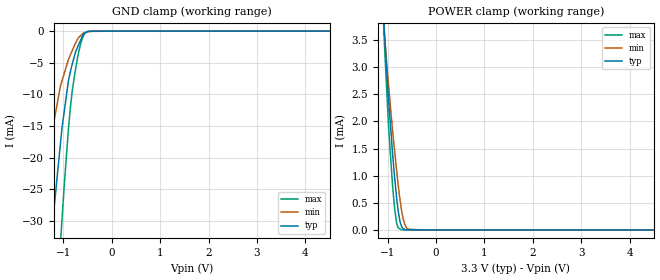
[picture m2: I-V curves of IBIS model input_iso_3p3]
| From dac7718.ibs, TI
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|   input_iso_3p3 Model
[Model]   input_iso_3p3
Model_type   Input
Vinl = 0.6
Vinh = 2.3
|   typ   min   max
|   (Nom PVT)   (Fast PVT)   (Slow PVT)
|C_comp from frequency method(F=50MHz)
|Average
|C_comp   3.924e-12   3.238e-12   4.430e-12
|C_comp from LC tank method(L=1nH)
|Resonant Frequency(Hz)   3.3e9   3.33e9   3.29e9
C_comp   2.328e-12   2.287e-12   2.343e-12
| Where nom  PVT is Nominal Process,  3.3V,  33C
|   Fast PVT is Strong Process,   3.6V,  -40C
|   Slow PVT is Weak Process,   3V,  113C
[Voltage Range]   3.3   3   3.6
|Ambient Temperature   25   85   -40
|Junction Temperature
[Temperature Range]   33   113   -40
[Power Clamp Reference]   3.3   3   3.6
[GND Clamp Reference]   0   0   0
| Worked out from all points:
|   GND clamp passes 1 mA (typ) near -0.62 V on its own axis
|   POWER clamp passes 1 mA (typ) near -0.86 V on its own axis
[GND Clamp]
|   Voltage   I(typ)   I(min)   I(max)
-3.3V     -263.7mA   -170.8mA   -345mA
-1.633V   -70.62mA   -38.28mA   -110.4mA
-1.476V   -54.49mA   -28.38mA   -88.21mA
-1.254V   -33.05mA   -16.57mA   -58.36mA
-1.204V   -28.72mA   -14.52mA   -51.84mA
-1.062V   -17.66mA   -8.638mA   -33.35mA
-1.033V   -15.41mA   -7.901mA   -29.97mA
-897.6mV  -7.809mA   -4.479mA   -15.45mA
-820.8mV  -5.258mA   -3.096mA   -9.571mA
-698.4mV  -2.347mA   -1.145mA   -3.782mA
-588mV    -438.4uA   -316uA     -761.5uA
6.6V      0A         0A         0A
[POWER Clamp]
|   Voltage   I(typ)   I(min)   I(max)
-3.3V     47.26mA    39.38mA    57.51mA
-1.092V   4.03mA     3.942mA    3.953mA
-1.066V   3.628mA    3.604mA    3.4mA
-982.8mV  2.421mA    2.68mA     1.915mA
-896.4mV  1.377mA    1.804mA    779.6uA
-853.2mV  934.2uA    1.429mA    369.8uA
-817.2mV  611.7uA    1.116mA    142.1uA
-778.8mV  326.4uA    799.1uA    36.82uA
-723.6mV  95.57uA    427.1uA    3.916uA
-645mV    7.29uA     97.76uA    2.834uA
-564mV    6.37uA     11.3uA     1.719uA
6.6V      0A         0A         0A
